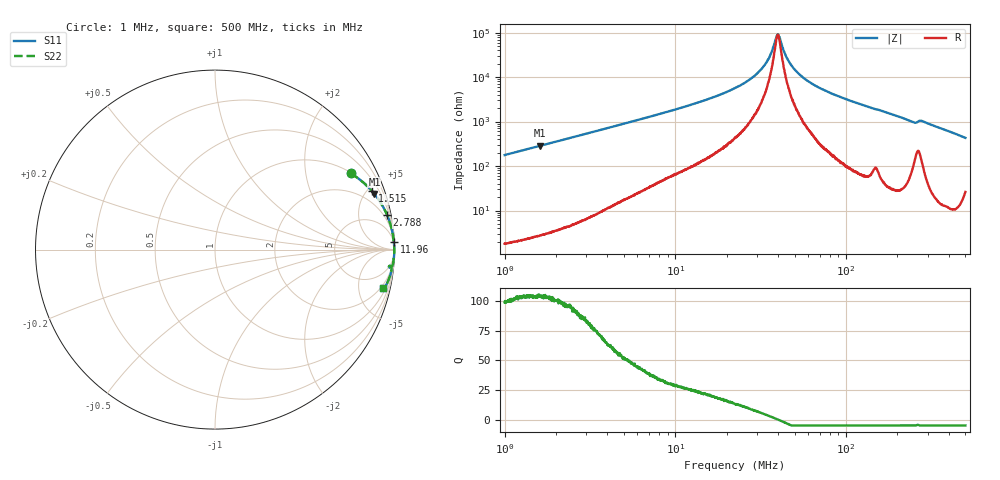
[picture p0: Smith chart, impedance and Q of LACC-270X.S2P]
!s-Parameter Generated by FASTRON Sdn. Bhd.
!FASTRON P/N : LACC-270X
!Keysight Technologies,E4991B,MY54100416,A.01.15
!Date: Wed Mar 18 09:41:03 2026
!Version  : Rev00 Wed Mar 18 09:41:03 2026
!Data & Calibration Information:
!PortZ  Port1:50+j0  Port2:50+j0
!When reading, reference impedance value at option line is always used.
!Remarks : This data is being provided solely for informational purposes.
!Freq	S11	S21	S12	S22
# Hz S dB R 50
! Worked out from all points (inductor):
!   1601 points, 1 MHz to 500 MHz, reference 50 ohm
!   read as one part in series: L = 28.1 uH near 1.032 MHz
!   highest Q = 105 at 1.612 MHz (marker M1), where L = 28.2 uH
!   self-resonance near 39.73 MHz
!   S11 on the Smith chart (normalised r, x): 1 MHz: 1.04, +3.54; 1.515 MHz: 1.05, +5.36; 2.788 MHz: 1.11, +9.90; 11.96 MHz: 3, +46; 500 MHz: 1.52, -8.59
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1000000  -1.24 29.4  -6.19 -60.1  -6.19 -60.1  -1.24 29.4
1515283  -0.59 20.4  -9.16 -69.1  -9.16 -69.1  -0.59 20.4
1612439  -0.53 19.3  -9.63 -70.2  -9.63 -70.2  -0.53 19.3
2788239  -0.19 11.4  -14.08 -78.0  -14.08 -78.0  -0.19 11.4
2820919  -0.19 11.3  -14.18 -78.1  -14.18 -78.1  -0.19 11.3
7957584  -0.04 3.9  -23.30 -84.4  -23.30 -84.4  -0.04 3.9
1.196468e7  -0.02 2.5  -27.26 -85.3  -27.26 -85.3  -0.02 2.5
2.236068e7  -0.01 1.0  -35.04 -84.7  -35.04 -84.7  -0.01 1.0
2.768612e7  -0.01 0.6  -39.33 -82.7  -39.33 -82.7  -0.01 0.6
3.233973e7  -0.01 0.3  -44.14 -78.8  -44.14 -78.8  -0.01 0.3
3.536177e7  -0.01 0.2  -48.72 -71.9  -48.72 -71.9  -0.01 0.2
3.88167e7  -0.01 0.0  -57.32 -33.5  -57.32 -33.5  -0.01 0.0
3.988656e7  -0.01 -0.0  -59.04 0.4  -59.04 0.4  -0.01 -0.0
4.098591e7  -0.01 -0.0  -57.44 36.6  -57.44 36.6  -0.01 -0.0
4.446912e7  -0.01 -0.2  -49.37 70.8  -49.37 70.8  -0.01 -0.2
4.806132e7  -0.01 -0.3  -45.10 78.8  -45.10 78.8  -0.01 -0.3
6.307767e7  -0.01 -0.8  -37.07 85.0  -37.07 85.0  -0.01 -0.8
9.265618e7  -0.01 -1.6  -31.03 86.5  -31.03 86.5  -0.01 -1.6
1.77937e8  -0.03 -3.7  -23.79 85.1  -23.79 85.1  -0.03 -3.7
2.475421e8  -0.14 -5.8  -19.81 78.2  -19.81 78.2  -0.14 -5.8
2.792168e8  -0.13 -5.5  -20.37 78.2  -20.37 78.2  -0.13 -5.5
5e8  -0.34 -12.9  -13.02 73.6  -13.02 73.6  -0.34 -12.9
